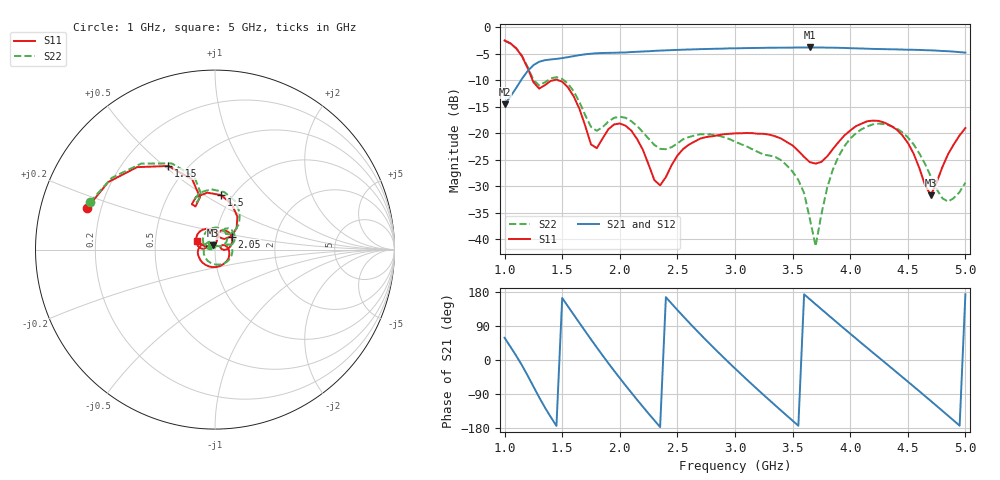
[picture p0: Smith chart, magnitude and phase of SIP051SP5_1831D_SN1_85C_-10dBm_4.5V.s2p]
# GHz  S  dB  R  50
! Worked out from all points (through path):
!   81 points, 1 GHz to 5 GHz, reference 50 ohm
!   highest |S21| = -3.83 dB at 3.65 GHz (marker M1); lowest = -14.5 dB at 1 GHz (marker M2)
!   lowest |S11| = -31.7 dB at 4.7 GHz (marker M3), VSWR 1.05, Z = 48.7 + j2.23 ohm
!   |S11| at or under -10 dB: 1.243 GHz to 1.428 GHz (185.3 MHz wide, 13.9 % of centre); 1.463 GHz to end of sweep
!   |S22| runs from -41.3 to -2.5 dB; largest |S21 - S12| = 0.0025
!   S11 on the Smith chart (normalised r, x): 1 GHz: 0.15, +0.16; 1.15 GHz: 0.40, +0.52; 1.5 GHz: 0.88, +0.59; 2.05 GHz: 1.19, +0.18; 5 GHz: 0.81, +0.08
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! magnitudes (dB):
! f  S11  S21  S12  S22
! 1 GHz  -2.5  -14.5  -14.5  -2.5
! 1.15 GHz  -5.5  -9.8  -9.8  -5.4
! 1.3 GHz  -11.6  -6.5  -6.5  -11.0
! 1.5 GHz  -10.3  -5.8  -5.8  -9.8
! 1.7 GHz  -18.6  -5.1  -5.1  -16.6
! 1.8 GHz  -22.8  -4.9  -4.9  -19.5
! 1.95 GHz  -18.3  -4.8  -4.8  -17.1
! 2.05 GHz  -18.6  -4.8  -4.8  -17.1
! 2.35 GHz  -29.8  -4.4  -4.4  -22.9
! 2.6 GHz  -22.1  -4.2  -4.2  -20.7
! 3 GHz  -20.0  -4.0  -4.0  -21.6
! 3.45 GHz  -21.7  -3.9  -3.9  -26.1
! 3.6 GHz  -24.5  -3.8  -3.8  -31.3
! 3.65 GHz  -25.4  -3.8  -3.8  -36.2
! 3.7 GHz  -25.7  -3.9  -3.8  -41.3
! 3.8 GHz  -24.4  -3.9  -3.9  -30.3
! 3.95 GHz  -20.4  -3.9  -3.9  -22.4
! 4.35 GHz  -18.6  -4.2  -4.2  -18.6
! 4.5 GHz  -21.8  -4.3  -4.2  -20.8
! 4.7 GHz  -31.7  -4.4  -4.4  -28.2
! 4.85 GHz  -23.9  -4.5  -4.6  -32.9
! 5 GHz  -19.0  -4.8  -4.8  -29.3
